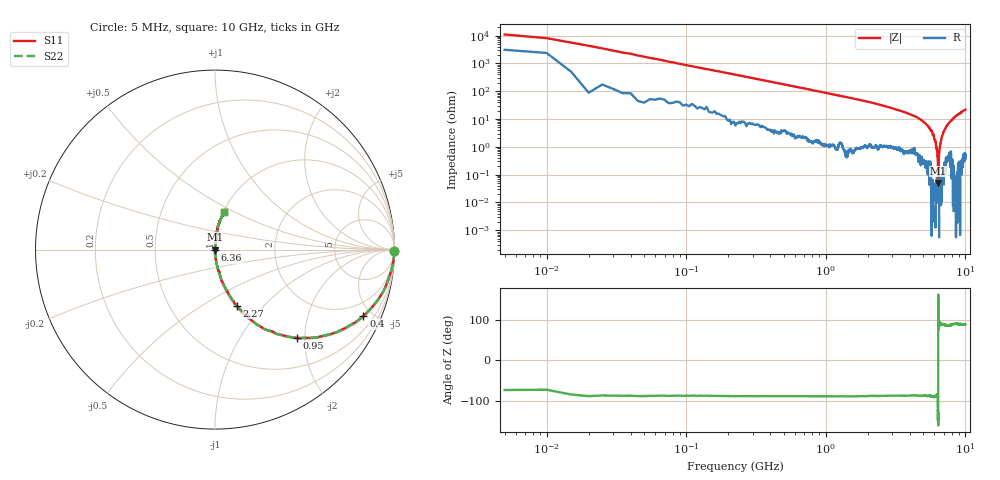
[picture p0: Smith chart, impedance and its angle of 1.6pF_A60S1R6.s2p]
! Amotech Co.,Ltd.
! http://www.amotech.co.kr/
! Part Number: A60S1R6
! These Parameters are Measured in Series Mode Connection
! Operation Temp=25[degC], DC Bias Voltage=0[V]
! Freq. Start=5[MHz] Stop=10[GHz], 2000[Steps]
! Date: Monday, July 13, 2020, 01:50:59
# GHZ S RI R 50.000000
!Freq.(Hz) S11(Real) S11(Imag) S21(Real) S21(Imag) S12(Real) S12(Imag) S22(Real) S22(Imag)
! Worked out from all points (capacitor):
!   2000 points, 5 MHz to 10 GHz, reference 50 ohm
!   read as one part in series: C = 1.83 pF near 55 MHz
!   lowest |Z| = 50.6 mohm at 6.405 GHz (marker M1)
!   series resonance near 6.388 GHz, so ESL is about 340 pH
!   S11 on the Smith chart (normalised r, x): 5 MHz: open; 400 MHz: 1.08, -4.44; 950 MHz: 1.03, -1.84; 2.27 GHz: 1.02, -0.72; 6.36 GHz: 1.00, -0.00; 10 GHz: 1.01, +0.44
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0.005  0.9974 -0.00869  0.00263 0.00869  0.00263 0.00869  0.9974 -0.00869
0.07  0.9905 -0.0793  0.00952 0.0793  0.00952 0.0793  0.9905 -0.0793
0.125  0.9746 -0.139  0.0254 0.139  0.0254 0.139  0.9746 -0.139
0.235  0.9302 -0.2457  0.0698 0.2457  0.0698 0.2457  0.9302 -0.2457
0.4  0.8266 -0.3694  0.1734 0.3694  0.1734 0.3694  0.8266 -0.3694
0.95  0.4577 -0.4912  0.5423 0.4912  0.5423 0.4912  0.4577 -0.4912
1.675  0.2105 -0.3991  0.7895 0.3991  0.7895 0.3991  0.2105 -0.3991
2.27  0.1222 -0.3126  0.8778 0.3126  0.8778 0.3126  0.1222 -0.3126
3.34  0.0489 -0.193  0.9511 0.193  0.9511 0.193  0.0489 -0.193
5.005  0.00945 -0.0791  0.9906 0.0791  0.9906 0.0791  0.00945 -0.0791
5.935  7.61e-06 -0.027  1 0.027  1 0.027  7.61e-06 -0.027
6.115  0.000308 -0.0155  0.9997 0.0155  0.9997 0.0155  0.000308 -0.0155
6.275  0.0007 -0.00714  0.9993 0.00714  0.9993 0.00714  0.0007 -0.00714
6.31  -2.87e-05 -0.00536  1 0.00536  1 0.00536  -2.87e-05 -0.00536
6.36  -0.00126 -0.000761  1.001 0.000761  1.001 0.000761  -0.00126 -0.000761
6.405  -0.000121 0.000491  1 -0.000491  1 -0.000491  -0.000121 0.000491
6.51  -0.00046 0.00664  1 -0.00664  1 -0.00664  -0.00046 0.00664
6.67  0.000425 0.0156  0.9996 -0.0156  0.9996 -0.0156  0.000425 0.0156
6.93  0.00193 0.0311  0.9981 -0.0311  0.9981 -0.0311  0.00193 0.0311
7.215  0.00476 0.0476  0.9952 -0.0476  0.9952 -0.0476  0.00476 0.0476
8.335  0.0123 0.1151  0.9877 -0.1151  0.9877 -0.1151  0.0123 0.1151
10  0.0494 0.2069  0.9506 -0.2069  0.9506 -0.2069  0.0494 0.2069
